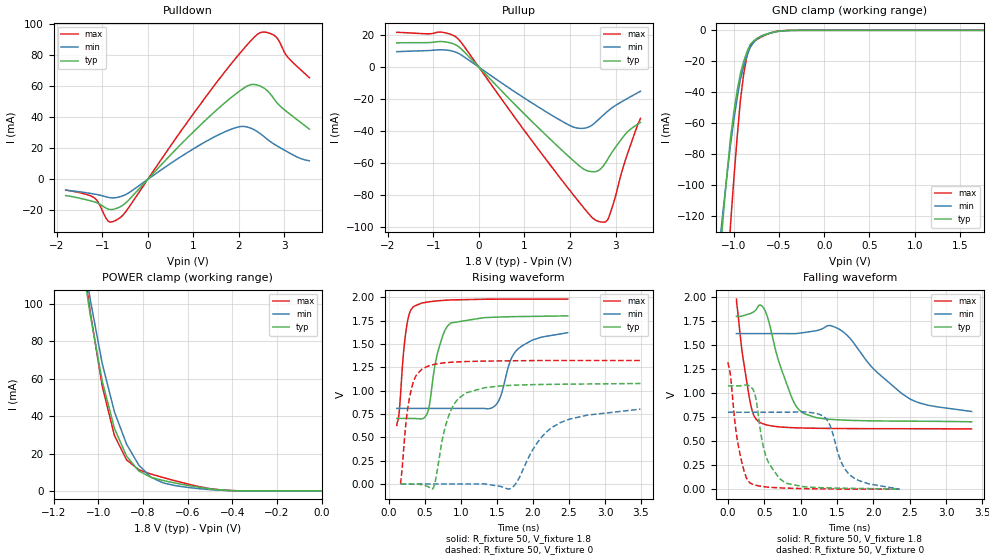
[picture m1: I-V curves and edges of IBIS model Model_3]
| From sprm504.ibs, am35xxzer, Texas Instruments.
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| Model based on original model for BC1833DV40CTPBFHP18LL_7LM
|   Sub model LL_7LM_PD_PU_OFF_1P8
[model]   Model_3
|[Description]  1.8V-I/O-PI-X
|[Input Load]   PI
|[Output Drive]
|Voltage   1.8V
|Mode   I/O
Model_type   I/O
Polarity   Non-Inverting
Enable   Active-Low
Vinl =  0.63V
Vinh =  1.17V
Cref =  15pF
Rref =  100.0000M
Vref =  0V
Vmeas =  0.9
C_comp   2.232809p   2.073051p   2.295852p
[Model Spec]
Vinl   0.63V   0.567V   0.693V
Vinh   1.17V   1.053V   1.287V
[Temperature Range]   25   125   -40
[Voltage Range]   1.8   1.62   1.98
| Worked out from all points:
|   slope of the pulldown table from 0 to 0.27 V, typ, clamps not added: 31.5 ohm
|   slope of the pullup table from 0 to 0.27 V, typ, clamps not added: 33.5 ohm
|   GND clamp passes 1 mA (typ) near -0.54 V on its own axis
|   POWER clamp passes 1 mA (typ) near -0.49 V on its own axis
|   rising waveform, R_fixture 50, V_fixture 1.8: 20-80 % time 168ps typ, 248ps min, 94.8ps max; typ from 0.702 V to 1.8 V
|   rising waveform, R_fixture 50, V_fixture 0: 20-80 % time 226ps typ, 478ps min, 132ps max; typ from 0 V to 1.08 V
|   falling waveform, R_fixture 50, V_fixture 1.8: 20-80 % time 283ps typ, 649ps min, 154ps max; typ from 1.8 V to 0.702 V
|   falling waveform, R_fixture 50, V_fixture 0: 20-80 % time 210ps typ, 246ps min, 145ps max; typ from 1.08 V to 0 V
[POWER_clamp]
-1.8V     842.2mA    869.1mA    912.5mA
-1.055V   109mA      116.8mA    112.5mA
-1.036V   94.63mA    102.8mA    96.22mA
-981.8mV  58.65mA    67.99mA    55.86mA
-927.3mV  33.42mA    42.23mA    29.64mA
-872.7mV  18.54mA    24.92mA    16.54mA
-818.2mV  10.66mA    13.77mA    11.33mA
-763.6mV  7.291mA    7.319mA    9.029mA
-709.1mV  5.568mA    4.279mA    7.154mA
-654.5mV  4.197mA    2.818mA    5.381mA
-436.4mV  381.9uA    275.7uA    348.1uA
0V        17.81nA    62.52nA    29.22nA
[Pulldown]
-1.8V     -10.48mA   -6.986mA   -6.871mA
-1.145V   -14.76mA   -9.635mA   -12.53mA
-872.7mV  -19.16mA   -11.57mA   -26.86mA
-600mV    -17.63mA   -11.14mA   -24.6mA
1.636V    48.02mA    29.94mA    67.34mA
2.073V    58.19mA    34.17mA    83.16mA
2.291V    61.26mA    32.65mA    90.37mA
2.455V    60.31mA    29.78mA    94.52mA
2.618V    57.35mA    25.94mA    94.79mA
2.782V    51.42mA    22.55mA    92.8mA
3.055V    43.58mA    17.93mA    79.45mA
3.545V    32.44mA    11.99mA    65.6mA
[Pullup]
-1.8V     15.25mA    9.689mA    21.84mA
-818.2mV  16.04mA    10.87mA    21.92mA
-490.9mV  13.71mA    9.212mA    18.64mA
1.036V    -30.4mA    -20.07mA   -41.09mA
2.018V    -57.11mA   -36.81mA   -77.94mA
2.345V    -64.48mA   -38.06mA   -89.56mA
2.618V    -64.84mA   -32.95mA   -96.49mA
2.782V    -59.78mA   -28.7mA    -96.85mA
2.836V    -57.13mA   -27.34mA   -95.02mA
3V        -50.06mA   -23.92mA   -80.63mA
3.218V    -41.82mA   -20.26mA   -57.92mA
3.545V    -34.58mA   -15.09mA   -32.06mA
[GND_clamp]
-1.8V     -697.8mA   -553.2mA   -1.259A
-1.145V   -140.6mA   -131.7mA   -248.3mA
-1.109V   -115.1mA   -111.6mA   -203.3mA
-1.036V   -69.6mA    -74.07mA   -125.9mA
-1V       -53.16mA   -58.25mA   -96.51mA
-927.3mV  -27.95mA   -31.85mA   -45.33mA
-890.9mV  -20.12mA   -23.33mA   -28.4mA
-854.5mV  -13.86mA   -16.38mA   -16.49mA
-818.2mV  -9.165mA   -11mA      -9.583mA
-745.5mV  -5.275mA   -5.606mA   -5.955mA
-418.2mV  -132.4uA   -214.4uA   -105.2uA
1.764V    17.27nA    517.3nA    24.83nA
[Ramp]
dV/dt_f  0.7278988/0.29621939n 0.53681274/0.67644425n 0.89199104/0.1621461n
dV/dt_r 0.67934265/0.22574009n  0.5133796/0.47382112n 0.81250299/0.13161562n
R_load = 50
[Rising Waveform]
R_fixture = 50
V_fixture = 1.8
V_fixture_min = 1.62
V_fixture_max = 1.98
106.5ps   701.7mV    809.2mV    626.9mV
140.6ps   701.7mV    809.2mV    780.1mV
238.5ps   701.7mV    809.2mV    1.665V
341.4ps   701.2mV    809.2mV    1.901V
536.5ps   768.6mV    809.2mV    1.949V
675ps     1.408V     809.2mV    1.961V
859.9ps   1.724V     809.2mV    1.971V
1.451ns   1.785V     824.9mV    1.979V
1.788ns   1.792V     1.444V     1.979V
2.482ns   1.8V       1.62V      1.98V
[Rising Waveform]
R_fixture = 50
V_fixture = 0
V_fixture_min = 0
V_fixture_max = 0
159.6ps   9.701nV    106.6nV    8.922nV
235.4ps   25.54uV    3.021uV    667.1mV
287.4ps   -398.5uV   2.15uV     941.3mV
459.5ps   -9.318mV   -415.9nV   1.231V
614.3ps   -40.83mV   2.575nV    1.278V
808ps     685.6mV    -1.409uV   1.3V
1.073ns   976mV      -266.7uV   1.311V
1.684ns   1.056V     -50.71mV   1.319V
2.269ns   1.067V     607.3mV    1.322V
3.493ns   1.076V     800.9mV    1.322V
[Falling Waveform]
R_fixture = 50
V_fixture = 1.8
V_fixture_min = 1.62
V_fixture_max = 1.98
116.9ps   1.8V       1.62V      1.98V
195.8ps   1.803V     1.62V      1.43V
304.1ps   1.829V     1.62V      915.6mV
446.2ps   1.916V     1.62V      693.6mV
541.2ps   1.8V       1.62V      667.8mV
864.7ps   979.6mV    1.62V      641mV
1.05ns    785.7mV    1.631V     636.7mV
1.479ns   723.6mV    1.686V     632mV
2.5ns     708mV      941.4mV    629.5mV
3.351ns   701.7mV    809.2mV    626.9mV
[Falling Waveform]
R_fixture = 50
V_fixture = 0
V_fixture_min = 0
V_fixture_max = 0
0s        1.076V     800.9mV    1.322V
147.4ps   1.075V     800.9mV    436.5mV
305.4ps   1.072V     800.9mV    65.08mV
375.8ps   973.8mV    800.9mV    42.61mV
469.1ps   507.8mV    800.9mV    28.31mV
533.7ps   320.1mV    800.9mV    22.37mV
794ps     62.3mV     800.9mV    10.93mV
1.296ns   15.02mV    766.5mV    2.927mV
1.661ns   9.448mV    160.8mV    1.006mV
2.364ns   9.701nV    106.6nV    8.922nV
